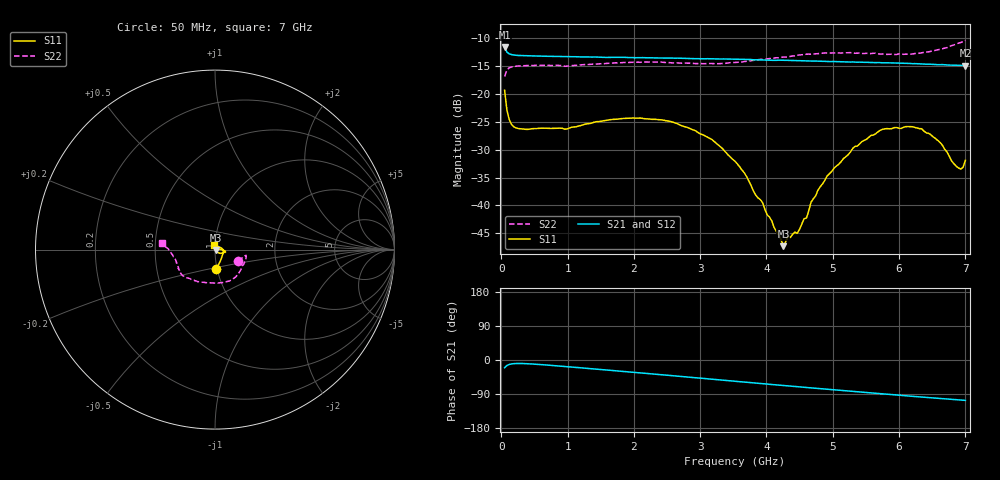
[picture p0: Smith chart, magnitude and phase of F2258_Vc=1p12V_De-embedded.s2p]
! Integrated Device Technology
! Corporate Headquarters
! 6024 Silver Creek Valley Road
! San Jose, CA 95138  USA
! Phone:  1-408-284-8200
! Toll Free:  1-800-223-1366
! Webpage:  http://www.idt.com/
! Timing and RF Division
! 515 Groton Road, Suite 102
! Westford, MA 01886-6024
! Device:  F2258
! Description: Voltage Variable RF Attenuator
! Frequency:  50.0 -  6000.00 MHz
! Package:  3x3 mm Thin QFN Plastic Package: 16 pin
! Ports:  2 RF, 2 DC
!  Pin  1  = NC
!  Pin  2  = NC
!  Pin  3  = RF2  = Port 2
!  Pin  4  = GND
!  Pin  5  = Vdd
!  Pin  6  = NC
!  Pin  7  = VCTRL
!  Pin  8  = NC
!  Pin  9  = GND
!  Pin 10  = RF1  = Port 1
!  Pin 11  = NC
!  Pin 12  = NC
!  Pin 13  = NC
!  Pin 14  = NC
!  Pin 15  = NC
!  Pin 16  = NC
! Vcntrl:  1.120 Volts
! Vdd:  +3.300 Volts
! Current:  1.162 mA
! Data:  The device was measured on a the F2258 evaluation board which has
!  individual transmission lines to the RF pins.  Data was collected
!  using a calibrated network analyzer.  The evaluation board was
!  de-embedded using a TRL calibration technique.
!  The reference plane is the edge of the package pin.
! Misc:  SN 10
!  Action Tracker AT0285
! Date Measured:  2014-12-10
! Date:  2016-01-13  MJV
! Note:
!  Integrated Device Technology supplies this data as a sample of measured
!  data at the package pin for this product.  Your particular data for this
!  product may vary.
!  Data was taken at 25 degrees C.
!  Integrated Device Technology reserves the right to change this data at anytime.
!Freq_(GHz)  S11M_(dB)  S11P_(deg)  S21M_(dB)  S21P_(deg)  S12M_(dB)  S12P_(deg)  S22M_(dB)  S22P_(deg)
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# GHz S dB R 50
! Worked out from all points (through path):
!   201 points, 50 MHz to 7 GHz, reference 50 ohm
!   highest |S21| = -11.63 dB at 50 MHz (marker M1); lowest = -15.0 dB at 7 GHz (marker M2)
!   group delay of S21, straight-line fit = 41 ps
!   lowest |S11| = -47.3 dB at 4.255 GHz (marker M3), VSWR 1.01, Z = 50.4 - j0.17 ohm
!   |S11| at or under -10 dB: start of sweep to end of sweep
!   |S22| runs from -16.9 to -10.4 dB; largest |S21 - S12| = 0.0015
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0.05  -19.36 -86.5  -11.63 -20.4  -11.58 -20.4  -16.91 -25.9
0.08475  -22.93 -66.0  -12.54 -14.6  -12.49 -14.5  -15.72 -14.4
0.1195  -24.62 -51.5  -12.84 -11.8  -12.80 -11.7  -15.34 -11.6
0.22375  -26.11 -30.6  -13.10 -9.3  -13.07 -9.2  -15.06 -10.7
1.2315  -25.57 -17.1  -13.40 -21.1  -13.35 -21.1  -14.79 -36.9
2.37825  -24.64 -9.0  -13.59 -38.3  -13.61 -38.3  -14.33 -65.6
3.1775  -28.20 -1.4  -13.74 -50.7  -13.74 -50.6  -14.60 -91.3
3.525  -32.09 2.4  -13.81 -56.1  -13.85 -56.1  -14.39 -104.9
3.942  -39.53 2.3  -13.94 -62.5  -13.95 -62.5  -13.85 -119.9
4.25475  -47.30 -23.0  -13.99 -67.3  -13.99 -67.3  -13.42 -129.1
4.32425  -45.50 -38.8  -14.01 -68.4  -14.03 -68.4  -13.41 -130.9
4.46325  -44.99 -56.3  -14.06 -70.5  -14.07 -70.5  -13.12 -134.5
4.60225  -42.27 -58.4  -14.12 -72.5  -14.10 -72.5  -12.91 -137.0
4.7065  -38.82 -54.4  -14.13 -74.1  -14.12 -74.1  -12.88 -138.8
4.915  -34.72 -49.4  -14.21 -77.2  -14.21 -77.2  -12.70 -141.8
5.332  -29.45 -35.6  -14.32 -83.3  -14.32 -83.2  -12.74 -147.9
5.85325  -26.28 -21.0  -14.46 -90.8  -14.46 -90.8  -12.92 -157.6
6.33975  -26.26 -5.6  -14.67 -97.8  -14.66 -97.9  -12.67 -169.7
6.61775  -28.71 14.9  -14.78 -101.6  -14.79 -101.6  -12.05 -177.5
6.89575  -33.30 69.1  -14.92 -105.3  -14.92 -105.3  -10.92 175.3
6.96525  -33.16 91.1  -14.95 -106.3  -14.96 -106.2  -10.65 173.9
7  -31.91 102.3  -14.97 -106.6  -14.97 -106.6  -10.45 173.0
